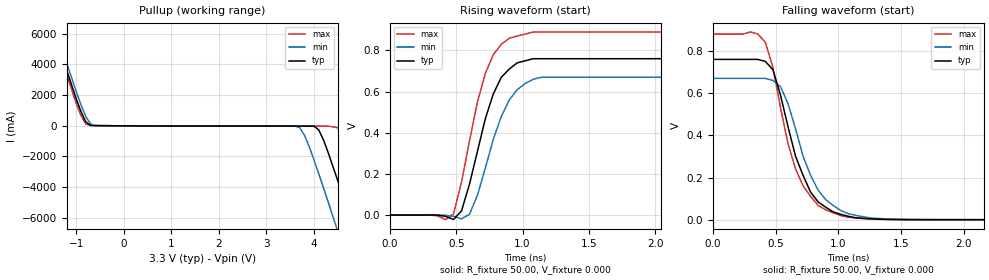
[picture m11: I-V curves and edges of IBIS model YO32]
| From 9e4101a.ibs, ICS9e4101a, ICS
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|   Model YO32
[Model]   YO32
Model_type   Open_source
Polarity   Inverting
C_comp   5.50pF   5.00pF   6.00pF
[Temperature Range]   27.00   70.00   0.000
[Voltage Range]   3.30V   3.00V   3.70V
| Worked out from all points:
|   slope of the pullup table from 0 to 0.495 V, typ, clamps not added: 56.2 ohm
|   rising waveform, R_fixture 50.00, V_fixture 0.000: 20-80 % time 193ps typ, 205ps min, 185ps max; typ from 0 V to 0.76 V
|   falling waveform, R_fixture 50.00, V_fixture 0.000: 20-80 % time 233ps typ, 241ps min, 223ps max; typ from 0.76 V to 0 V
[Pullup]
| voltage   I(typ)   I(min)   I(max)
-3.3V     24.07A     24.5A      23.8A
-1.5V     6.41A      6.88A      6.12A
-1V       1.75A      2.22A      1.46A
-800mV    260mA      610mA      110mA
-600mV    14.66mA    17.87mA    15.76mA
3.7V      -15.26mA   -120mA     -17.76mA
4.1V      -260mA     -3.12A     -17.79mA
4.5V      -3.57A     -6.88A     -120mA
4.7V      -5.46A     -8.81A     -1.47A
4.9V      -7.39A     -10.75A    -3.28A
5.3V      -11.28A    -14.66A    -7.1A
6.6V      -24.09A    -27.49A    -19.87A
[Ramp]
| variable   typ   min   max
dV/dt_r   0.46/0.19n   0.40/0.20n   0.53/0.18n
dV/dt_f   0.45/0.23n   0.40/0.24n   0.53/0.22n
R_load = 50.00
[Rising Waveform]
R_fixture = 50.00
V_fixture = 0.000
V_fixture_min = 0.000
V_fixture_max = 0.000
| time   V(typ)   V(min)   V(max)
0s        -29.01uV   -27.14uV   -30.44uV
420ps     -6.28mV    -800uV     -22.42mV
480ps     -21.47mV   -5.82mV    6.3mV
540ps     20.11mV    -18.37mV   160mV
600ps     150mV      3.85mV     360mV
720ps     470mV      230mV      690mV
840ps     670mV      480mV      830mV
900ps     710mV      560mV      860mV
1.14ns    760mV      670mV      890mV
3ns       760mV      670mV      880mV
[Falling Waveform]
R_fixture = 50.00
V_fixture = 0.000
V_fixture_min = 0.000
V_fixture_max = 0.000
| time   V(typ)   V(min)   V(max)
0s        760mV      670mV      880mV
300ps     760mV      670mV      890mV
420ps     750mV      670mV      840mV
480ps     710mV      660mV      720mV
540ps     590mV      630mV      530mV
660ps     300mV      430mV      240mV
780ps     130mV      210mV      110mV
900ps     59.13mV    95.22mV    46.83mV
1.26ns    4.41mV     8.08mV     3.03mV
3ns       -16.33uV   4.91uV     4.26uV
